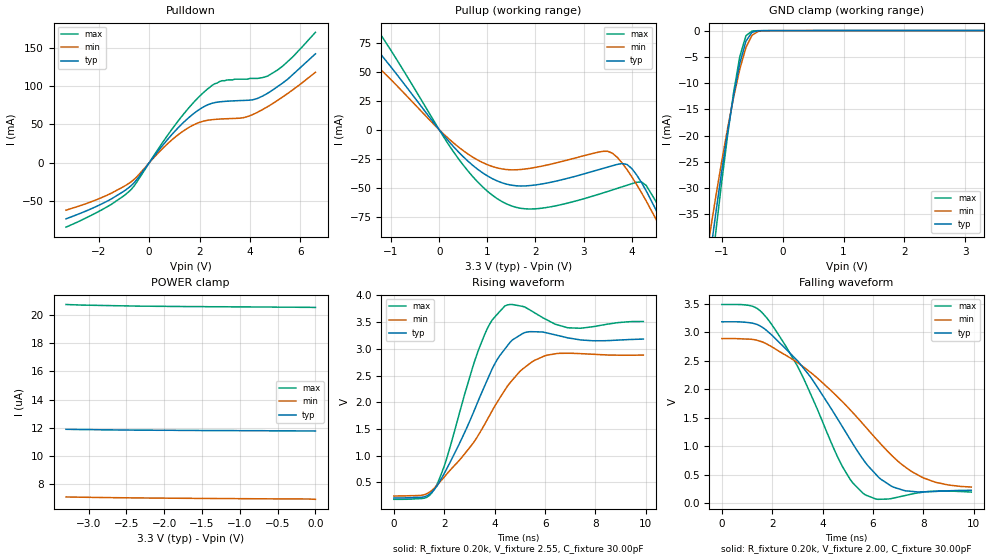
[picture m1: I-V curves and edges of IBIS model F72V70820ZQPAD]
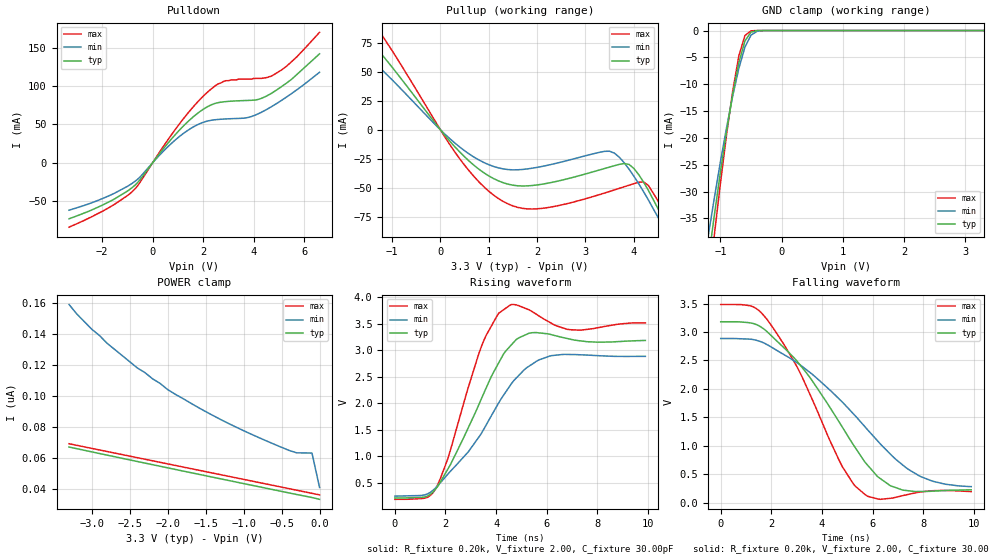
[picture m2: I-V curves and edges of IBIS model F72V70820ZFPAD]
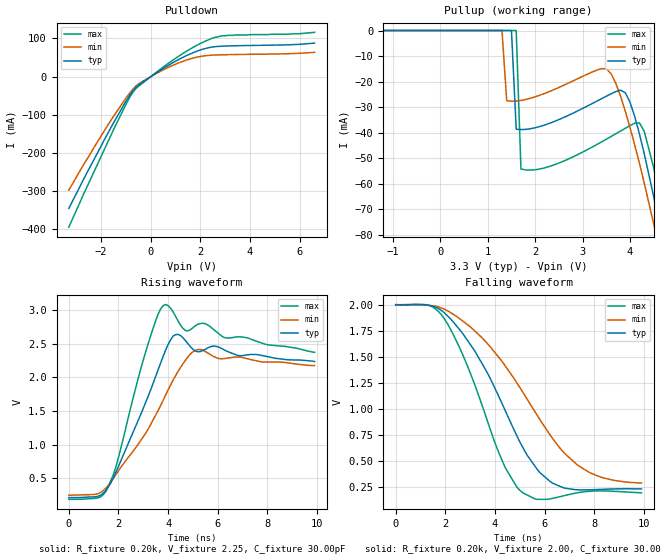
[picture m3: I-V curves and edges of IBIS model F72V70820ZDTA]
| IBIS file 72V70200.ibs manually created by editing orignal
| IBIS file f72v7082.ibs created by s2ibis2 version 1.1
| North Carolina State University Electronics Research Laboratory  1995
[IBIS ver]   2.1
[File name]   72v70200.ibs
[File Rev]   1.0
[Date]   03/06/2012
[Source]   Integrated Device Technology, Inc.
[Notes]   1. Temperatures: typ=25C, min=85C, max=-40C 2. Cemos9_3v
   process. 3. Ramp rates based on 50 ohm load.
[Disclaimer] Integrated Device Technology, Inc. ("IDT") hereby grants the
   user of this IBIS model a non-exclusive, nontransferable
   license to use this IBIS model under the following terms. The
   user is granted this license only to use the IBIS model and is
   not granted rights to sell, copy (except as needed to run the
   IBIS model), rent, lease or sub-license the IBIS model in
   whole or in part, or in modified form to anyone. The User may
   modify the IBIS model to suit its specific applications, but
   rights to derivative works and such modifications shall belong
   to IDT. This IBIS model is provided on an AS IS" basis and IDT
   makes absolutely no warranty with respect to the information
   contained herein. IDT DISCLAIMS AND CUSTOMER WAIVES ALL
   WARRANTIES, EXPRESS AND IMPLIED, INCLUDING WARRANTIES OF
   MERCHANTABILITY AND FITNESS FOR A PARTICULAR PURPOSE. THE
   ENTIRE RISK AS TO QUALITY AND PERFORMANCE IS WITH THE USER
   ACCORDINGLY, IN NO EVENT SHALL IDT BE LIABLE FOR ANY DIRECT OR
   INDIRECT DAMAGES, WHETHER IN CONTRACT OR TORT, INCLUDING ANY
   LOST PROFITS OR OTHER INCIDENTAL, CONSEQUENTIAL, EXEMPLARY, OR
   PUNITIVE DAMAGES ARISING OUT OF THE USE OR APPLICATION OF THE
   IBIS model. Further, IDT reserves the right to make changes
   without notice to any product herein to improve reliability,
   function, or design. IDT does not convey any license under
   patent rights or any other intellectual property rights,
   including those of third parties. IDT is not obligated to
   provide maintenance or support for the licensed IBIS model.
[Copyright]   Copyright 1999,2000,2012, Integrated Device Technology, Inc.
   all rights reserved
|   Component idt72v70200
[Component]   idt72v70200
[Manufacturer]   Integrated Device Technology
[Package]
| TQFP(PN100)
| variable   typ   min   max
R_pkg   10.00m   9.00m   11.00m
L_pkg   4.50nH   4.10nH   5.10nH
C_pkg   0.16pF   0.11pF   0.22pF
[Pin]  signal_name   model_name   R_pin   L_pin   C_pin
3   TMS   F72V70820ZTTLPU
4   TDI   F72V70820ZTTLPU
5   TDO   F72V70820ZFPAD
6   TCK   F72V70820ZTTL
7   TRST   F72V70820ZTTLU2
8   IC   F72V70820ZTTLPD
9   RESET   F72V70820ZTTL
10   IC   F72V70820ZTTL
11   A0   F72V70820ZTTL
12   A1   F72V70820ZTTL
13   A2   F72V70820ZTTL
14   A3   F72V70820ZTTL
15   A4   F72V70820ZTTL
16   A5   F72V70820ZTTL
17   A6   F72V70820ZTTL
18   A7   F72V70820ZTTL
19   DS_RD   F72V70820ZTTL
20   R_W_RW   F72V70820ZTTL
21   CS   F72V70820ZTTL
22   AS_ALE   F72V70820ZTTL
23   IM   F72V70820ZTTL
28   GND   GND
29   AD0   F72V70820ZQPAD
30   AD1   F72V70820ZQPAD
31   AD2   F72V70820ZQPAD
32   AD3   F72V70820ZQPAD
33   AD4   F72V70820ZQPAD
34   AD5   F72V70820ZQPAD
35   AD6   F72V70820ZQPAD
36   AD7   F72V70820ZQPAD
37   VCC   POWER
38   GND   GND
39   D8   F72V70820ZQPAD
40   D9   F72V70820ZQPAD
41   D10   F72V70820ZQPAD
42   D11   F72V70820ZQPAD
43   D12   F72V70820ZQPAD
44   D13   F72V70820ZQPAD
45   D14   F72V70820ZQPAD
46   D15   F72V70820ZQPAD
47   DTA   F72V70820ZDTA
48   CCO   F72V70820ZFPAD
53   GND   GND
54   ODE   F72V70820ZTTL
55   TX0   F72V70820ZFPAD
56   TX1   F72V70820ZFPAD
57   TX2   F72V70820ZFPAD
58   TX3   F72V70820ZFPAD
59   TX4   F72V70820ZFPAD
60   TX5   F72V70820ZFPAD
61   TX6   F72V70820ZFPAD
62   TX7   F72V70820ZFPAD
63   GND   GND
64   VCC   POWER
65   TX8   F72V70820ZFPAD
66   TX9   F72V70820ZFPAD
67   TX10   F72V70820ZFPAD
68   TX11   F72V70820ZFPAD
69   TX12   F72V70820ZFPAD
70   TX13   F72V70820ZFPAD
71   TX14   F72V70820ZFPAD
72   TX15   F72V70820ZFPAD
73   GND   GND
78   RX0   F72V70820ZTTL2
79   RX1   F72V70820ZTTL2
80   RX2   F72V70820ZTTL2
81   RX3   F72V70820ZTTL2
82   RX4   F72V70820ZTTL2
83   RX5   F72V70820ZTTL2
84   RX6   F72V70820ZTTL2
85   RX7   F72V70820ZTTL2
86   RX8   F72V70820ZTTL2
87   RX9   F72V70820ZTTL2
88   RX10   F72V70820ZTTL2
89   RX11   F72V70820ZTTL2
90   RX12   F72V70820ZTTL2
91   RX13   F72V70820ZTTL2
92   RX14   F72V70820ZTTL2
93   RX15   F72V70820ZTTL2
94   F0I   F72V70820ZTTL
95   FE_HCLK   F72V70820ZTTL
96   GND   GND
97   CLK   F72V70820ZTTL
98   VCC   POWER
| Models and submodels in the file (8): F72V70820ZQPAD (I/O), F72V70820ZFPAD (3-state), F72V70820ZDTA (Output), F72V70820ZTTL (Input), F72V70820ZTTL2 (Input), F72V70820ZTTLPU (Input), F72V70820ZTTLU2 (Input), F72V70820ZTTLPD (Input)
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| FIN  FIN   dummy_model
| FOEL FOEL   dummy_model
| QIN  QIN   dummy_model
| QOEL QOEL   dummy_model
| DIN  DIN   dummy_model
|   Model F72V70820ZQPAD
[Model]   F72V70820ZQPAD
Model_type   I/O
Polarity   Non-Inverting
Enable   Active-Low
Vinl =  0.000V
Vinh =  3.000V
Vmeas =  1.500V
C_comp   3.00pF   NA   NA
[Temperature Range]   25.00   85.00   -40.00
[Voltage Range]   3.30V   3.00V   3.60V
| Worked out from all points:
|   slope of the pulldown table from 0 to 0.495 V, typ, clamps not added: 23.4 ohm
|   slope of the pullup table from 0 to 0.495 V, typ, clamps not added: 21.5 ohm
|   GND clamp passes 1 mA (typ) near -0.54 V on its own axis
|   rising waveform, R_fixture 0.20k, V_fixture 2.55, C_fixture 30.00pF: 20-80 % time 1.71ns typ, 2.27ns min, 1.23ns max; typ from 0.211 V to 3.18 V
|   falling waveform, R_fixture 0.20k, V_fixture 2.00, C_fixture 30.00pF: 20-80 % time 2.73ns typ, 3.51ns min, 2.12ns max; typ from 3.18 V to 0.229 V
[Pulldown]
| voltage   I(typ)   I(min)   I(max)
-3.3V     -72.9mA    -61.6mA    -83.7mA
-1.7V     -50.47mA   -42.52mA   -57.8mA
-800mV    -32mA      -26.54mA   -37.34mA
1.2V      47.35mA    37.83mA    56.6mA
1.9V      67.47mA    51.48mA    83.41mA
2.5V      77.67mA    56.26mA    101mA
2.9V      79.81mA    57.22mA    107mA
3.8V      81.36mA    59.3mA     109mA
4.2V      82.85mA    64.29mA    110mA
4.7V      90.6mA     73.15mA    113mA
5.3V      104mA      85.84mA    126mA
6.6V      142mA      118mA      170mA
[Pullup]
| voltage   I(typ)   I(min)   I(max)
-3.3V     146mA      105mA      190mA
-2.3V     116mA      90.88mA    147mA
-1.5V     79.72mA    63.5mA     100mA
-1V       53.96mA    43.07mA    68.21mA
400mV     -19.13mA   -14.87mA   -24.99mA
1.4V      -46.88mA   -34.3mA    -63.9mA
3.5V      -32.14mA   -18.54mA   -53.16mA
3.9V      -29.89mA   -34.29mA   -47.81mA
4.2V      -45.33mA   -54.06mA   -44.96mA
4.7V      -86.48mA   -93.01mA   -79.56mA
4.9V      -105mA     -110mA     -99.7mA
6.6V      -284mA     -270mA     -297mA
[GND_clamp]
| voltage   I(typ)   I(min)   I(max)
-3.3V     -263mA     -228mA     -298mA
-1.2V     -43.96mA   -39.28mA   -49.29mA
-1.1V     -35.25mA   -32mA      -38.93mA
-1V       -26.98mA   -25.08mA   -29.06mA
-900mV    -19.24mA   -18.57mA   -19.87mA
-800mV    -12.2mA    -12.56mA   -11.61mA
-700mV    -6.204mA   -7.29mA    -4.893mA
-600mV    -2.013mA   -3.2mA     -972uA
-500mV    -309uA     -878uA     -70.72uA
-400mV    -29.78uA   -143uA     -9.346uA
-300mV    -4.901uA   -18.95uA   -5.393uA
3.3V      11.76uA    6.916uA    20.55uA
[POWER_clamp]
| voltage   I(typ)   I(min)   I(max)
-3.3V     11.88uA    7.059uA    20.77uA
-3.1V     11.86uA    7.041uA    20.73uA
-2.3V     11.82uA    6.988uA    20.65uA
-1.7V     11.8uA     6.962uA    20.62uA
-1.5V     11.79uA    6.954uA    20.62uA
-1.1V     11.79uA    6.941uA    20.6uA
-1V       11.78uA    6.938uA    20.6uA
-700mV    11.78uA    6.928uA    20.59uA
-600mV    11.77uA    6.925uA    20.59uA
-500mV    11.77uA    6.922uA    20.58uA
-100mV    11.76uA    6.914uA    20.57uA
0V        11.76uA    6.89uA     20.56uA
[Ramp]
| variable   typ   min   max
dV/dt_r   1.29/1.36n   1.01/2.25n   1.57/0.87n
dV/dt_f   1.28/3.10n   1.01/4.05n   1.50/2.20n
R_load = 50.00
[Rising Waveform]
R_fixture = 0.20k
V_fixture = 2.55
C_fixture = 30.00pF
R_dut = 0.75
L_dut = 8.10nH
C_dut = 0.53pF
| time   V(typ)   V(min)   V(max)
0s        211mV      247mV      185mV
1.6ns     371mV      393mV      367mV
2ns       672mV      605mV      808mV
3.4ns     2.089V     1.424V     3.032V
3.9ns     2.626V     1.842V     3.539V
4.4ns     2.994V     2.226V     3.801V
5.2ns     3.305V     2.655V     3.78V
6.1ns     3.294V     2.883V     3.535V
7.4ns     3.167V     2.91V      3.385V
9.9ns     3.182V     2.882V     3.511V
[Falling Waveform]
R_fixture = 0.20k
V_fixture = 2.00
C_fixture = 30.00pF
R_dut = 0.75
L_dut = 8.10nH
C_dut = 0.53pF
| time   V(typ)   V(min)   V(max)
0s        3.18V      2.886V     3.483V
1.2ns     3.158V     2.873V     3.455V
1.9ns     2.98V      2.763V     3.182V
3.5ns     2.225V     2.301V     1.938V
4.8ns     1.331V     1.775V     634mV
5.6ns     775mV      1.392V     178mV
6.3ns     426mV      1.044V     72.11mV
7.2ns     229mV      663mV      130mV
8.5ns     209mV      367mV      215mV
9.9ns     229mV      286mV      198mV
|   Model F72V70820ZFPAD
[Model]   F72V70820ZFPAD
Model_type   3-state
Polarity   Non-Inverting
Enable   Active-Low
Vinl =  0.000V
Vinh =  3.000V
Vmeas =  1.500V
C_comp   3.00pF   NA   NA
[Temperature Range]   25.00   85.00   -40.00
[Voltage Range]   3.30V   3.00V   3.60V
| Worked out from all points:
|   slope of the pulldown table from 0 to 0.495 V, typ, clamps not added: 23.4 ohm
|   slope of the pullup table from 0 to 0.495 V, typ, clamps not added: 21.5 ohm
|   GND clamp passes 1 mA (typ) near -0.54 V on its own axis
|   rising waveform, R_fixture 0.20k, V_fixture 2.00, C_fixture 30.00pF: 20-80 % time 1.75ns typ, 2.28ns min, 1.25ns max; typ from 0.211 V to 3.18 V
|   falling waveform, R_fixture 0.20k, V_fixture 2.00, C_fixture 30.00pF: 20-80 % time 2.74ns typ, 3.51ns min, 2.14ns max; typ from 3.18 V to 0.229 V
[Pulldown]
| voltage   I(typ)   I(min)   I(max)
-3.3V     -72.8mA    -61.6mA    -83.7mA
-1.9V     -53.7mA    -45.35mA   -61.6mA
-800mV    -32.01mA   -26.54mA   -37.34mA
1.2V      47.36mA    37.84mA    56.62mA
1.9V      67.48mA    51.49mA    83.43mA
2.5V      77.68mA    56.27mA    101mA
2.9V      79.82mA    57.23mA    107mA
3.8V      81.36mA    59.3mA     109mA
4.2V      82.85mA    64.29mA    110mA
4.7V      90.6mA     73.15mA    113mA
5.3V      104mA      85.84mA    126mA
6.6V      142mA      118mA      170mA
[Pullup]
| voltage   I(typ)   I(min)   I(max)
-3.3V     146mA      106mA      190mA
-2.3V     116mA      90.89mA    147mA
-1.5V     79.73mA    63.51mA    100mA
-1V       53.97mA    43.08mA    68.23mA
400mV     -19.13mA   -14.87mA   -24.99mA
1.4V      -46.88mA   -34.3mA    -63.9mA
3.5V      -32.14mA   -18.51mA   -53.16mA
3.9V      -29.82mA   -33.81mA   -47.81mA
4.2V      -44.86mA   -53.11mA   -44.92mA
4.7V      -85.13mA   -91.19mA   -78.74mA
4.9V      -103mA     -108mA     -98.49mA
6.6V      -279mA     -265mA     -292mA
[GND_clamp]
| voltage   I(typ)   I(min)   I(max)
-3.3V     -257mA     -223mA     -293mA
-1.2V     -42.98mA   -38.32mA   -48.28mA
-1.1V     -34.44mA   -31.21mA   -38.11mA
-1V       -26.34mA   -24.44mA   -28.43mA
-900mV    -18.77mA   -18.08mA   -19.41mA
-800mV    -11.88mA   -12.22mA   -11.32mA
-700mV    -6.026mA   -7.079mA   -4.749mA
-600mV    -1.941mA   -3.095mA   -929uA
-500mV    -292uA     -843uA     -59.24uA
-400mV    -24.21uA   -135uA     -2.053uA
-300mV    -1.458uA   -16.11uA   -49.02nA
3.3V      33.11nA    63.46nA    33nA
[POWER_clamp]
| voltage   I(typ)   I(min)   I(max)
-3.3V     66.92nA    159nA      69.05nA
-3.2V     65.88nA    153nA      68.04nA
-3V       63.79nA    143nA      66.04nA
-2.9V     62.75nA    139nA      65.04nA
-2.8V     61.71nA    134nA      64.04nA
-2.4V     57.58nA    118nA      60.04nA
-1.9V     52.45nA    101nA      55.03nA
-1.3V     46.35nA    84.64nA    49.03nA
-700mV    40.28nA    70.88nA    43.02nA
-300mV    36.24nA    63.16nA    39.02nA
-100mV    34.31nA    63.03nA    37.01nA
0V        33.14nA    40.81nA    36.01nA
[Ramp]
| variable   typ   min   max
dV/dt_r   1.29/1.37n   1.01/2.24n   1.57/0.93n
dV/dt_f   1.28/3.10n   1.01/4.05n   1.50/2.21n
R_load = 50.00
[Rising Waveform]
R_fixture = 0.20k
V_fixture = 2.00
C_fixture = 30.00pF
R_dut = 0.75
L_dut = 8.10nH
C_dut = 0.53pF
| time   V(typ)   V(min)   V(max)
0s        211mV      247mV      185mV
1.6ns     375mV      396mV      376mV
2.1ns     761mV      664mV      962mV
3.5ns     2.171V     1.496V     3.163V
4.1ns     2.757V     2.003V     3.694V
4.5ns     3.044V     2.293V     3.831V
5.3ns     3.318V     2.696V     3.76V
6.2ns     3.289V     2.896V     3.502V
7.3ns     3.176V     2.912V     3.376V
9.9ns     3.182V     2.882V     3.513V
[Falling Waveform]
R_fixture = 0.20k
V_fixture = 2.00
C_fixture = 30.00pF
R_dut = 0.75
L_dut = 8.10nH
C_dut = 0.53pF
| time   V(typ)   V(min)   V(max)
0s        3.18V      2.886V     3.483V
1.2ns     3.158V     2.873V     3.455V
1.8ns     3.019V     2.786V     3.239V
3.1ns     2.441V     2.436V     2.316V
4.8ns     1.335V     1.772V     640mV
5.3ns     981mV      1.536V     300mV
5.7ns     716mV      1.337V     148mV
6.7ns     302mV      858mV      80.16mV
7.8ns     200mV      486mV      185mV
9.9ns     229mV      285mV      198mV
|   Model F72V70820ZDTA
[Model]   F72V70820ZDTA
Model_type   Output
Vmeas =  1.500V
C_comp   3.00pF   NA   NA
[Temperature Range]   25.00   85.00   -40.00
[Voltage Range]   3.30V   3.00V   3.60V
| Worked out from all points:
|   slope of the pulldown table from 0 to 0.495 V, typ, clamps not added: 23.4 ohm
|   rising waveform, R_fixture 0.20k, V_fixture 2.25, C_fixture 30.00pF: 20-80 % time 1.39ns typ, 1.93ns min, 902ps max; typ from 0.211 V to 2.23 V
|   falling waveform, R_fixture 0.20k, V_fixture 2.00, C_fixture 30.00pF: 20-80 % time 2.3ns typ, 3.02ns min, 1.73ns max; typ from 2 V to 0.227 V
[Pulldown]
| voltage   I(typ)   I(min)   I(max)
-3.3V     -345mA     -297mA     -394mA
-1.7V     -145mA     -124mA     -167mA
-1V       -64.57mA   -56.38mA   -72.75mA
-700mV    -35.55mA   -31.63mA   -39.13mA
-500mV    -22.44mA   -19.4mA    -25.6mA
400mV     17.24mA    14.26mA    20.09mA
1.2V      47.36mA    37.84mA    56.62mA
2V        69.73mA    52.76mA    86.75mA
2.6V      78.47mA    56.58mA    103mA
3.4V      80.84mA    57.89mA    109mA
5.5V      83.3mA     59.95mA    111mA
6.6V      87.77mA    63.64mA    116mA
[Pullup]
| voltage   I(typ)   I(min)   I(max)
-3.3V     66.93nA    154nA      70.31nA
1.3V      20.09nA    25nA       23.2nA
1.4V      19.09nA    -27.44mA   22.17nA
1.5V      18.09nA    -27.64mA   21.15nA
1.6V      -38.62mA   -27.6mA    20.12nA
1.7V      -38.76mA   -27.36mA   -54.17mA
3.4V      -26.67mA   -14.9mA    -43.57mA
3.8V      -23.33mA   -25.71mA   -39.32mA
4.2V      -40.6mA    -52.13mA   -36.17mA
4.5V      -65.11mA   -75.73mA   -53.81mA
4.9V      -103mA     -110mA     -93.8mA
6.6V      -289mA     -277mA     -300mA
[Ramp]
| variable   typ   min   max
dV/dt_r   1.11/1.39n   0.83/2.31n   1.38/0.89n
dV/dt_f   1.28/3.11n   1.01/4.06n   1.51/2.22n
R_load = 50.00
[Rising Waveform]
R_fixture = 0.20k
V_fixture = 2.25
C_fixture = 30.00pF
R_dut = 0.75
L_dut = 8.10nH
C_dut = 0.53pF
| time   V(typ)   V(min)   V(max)
0s        211mV      247mV      185mV
1.5ns     320mV      352mV      307mV
1.9ns     591mV      554mV      671mV
3.2ns     1.721V     1.231V     2.503V
3.8ns     2.311V     1.659V     3.065V
4.4ns     2.638V     2.087V     2.838V
4.7ns     2.545V     2.255V     2.694V
5.2ns     2.379V     2.413V     2.788V
5.9ns     2.462V     2.298V     2.69V
9.9ns     2.235V     2.174V     2.371V
[Falling Waveform]
R_fixture = 0.20k
V_fixture = 2.00
C_fixture = 30.00pF
R_dut = 0.75
L_dut = 8.10nH
C_dut = 0.53pF
| time   V(typ)   V(min)   V(max)
0s        2V         2V         2V
1.3ns     1.996V     1.997V     1.997V
1.9ns     1.934V     1.963V     1.885V
3.2ns     1.549V     1.743V     1.22V
4.4ns     988mV      1.415V     438mV
5.1ns     635mV      1.166V     194mV
6.2ns     303mV      754mV      130mV
7.3ns     219mV      461mV      189mV
8.4ns     224mV      331mV      207mV
9.9ns     227mV      283mV      190mV
